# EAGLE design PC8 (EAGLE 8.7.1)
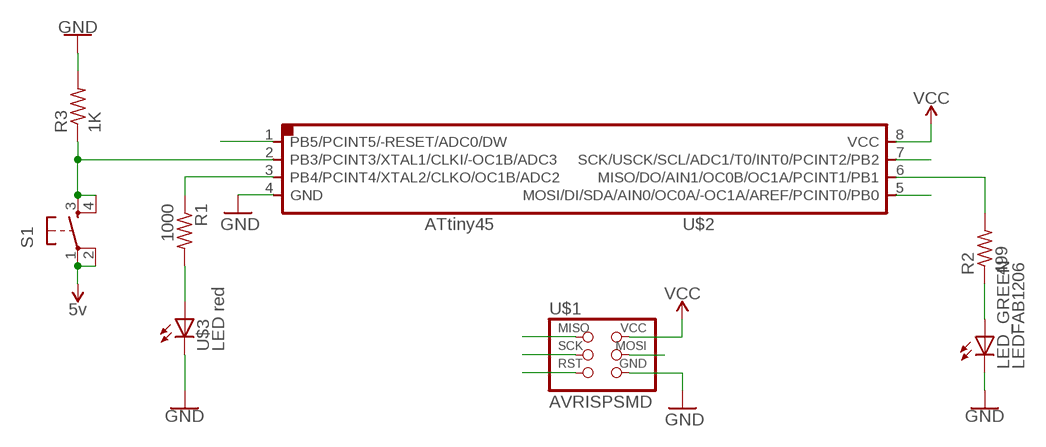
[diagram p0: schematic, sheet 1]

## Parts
LED_GREEN  LEDFAB1206  [LED1206FAB]
R1  1000  RES-US1206FAB  [R1206FAB]
R2  499  RES-US1206FAB  [R1206FAB]
R3  1K  RES-US1206FAB  [R1206FAB]
S1  6MM_SWITCH6MM_SWITCH  [6MM_SWITCH]
U$1  AVRISPSMD  [2X03SMD]
U$2  ATTINY45SI  [SOIC8]
U$3  LED red  LEDFAB1206  [LED1206FAB]

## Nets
GND: LED_GREEN.2(C) R3.2 U$1.6(GND) U$2.4(GND) U$3.2(C)
MISO: R2.2 U$1.1(MISO) U$2.6(MISO/DO/AIN1/OC0B/OC1A/PCINT1/PB1)
MOSI: U$1.4(MOSI) U$2.5(MOSI/DI/SDA/AIN0/OC0A/-OC1A/AREF/PCINT0/PB0)
N$1: R3.1 S1.3(S) S1.4(S1) U$2.2(PB3/PCINT3/XTAL1/CLKI/-OC1B/ADC3)
N$2: R1.1 U$2.3(PB4/PCINT4/XTAL2/CLKO/OC1B/ADC2)
N$3: R1.2 U$3.1(A)
N$4: LED_GREEN.1(A) R2.1
RST: U$1.5(RST) U$2.1(PB5/PCINT5/-RESET/ADC0/DW)
SCK: U$1.3(SCK) U$2.7(SCK/USCK/SCL/ADC1/T0/INT0/PCINT2/PB2)
VCC: S1.1(P) S1.2(P1) U$1.2(VCC) U$2.8(VCC) ; supply symbol labelled 5v

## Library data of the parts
LED_GREEN U$3 = fab (1):LED: LED
R1 R2 = fab:RES-US: Resistor (US Symbol)
R3 = fab (1):RES-US: Resistor (US Symbol)
S1 = fab:6MM_SWITCH: OMRON SWITCH
U$1 = fab:AVRISP
U$2 = fab:ATTINY45

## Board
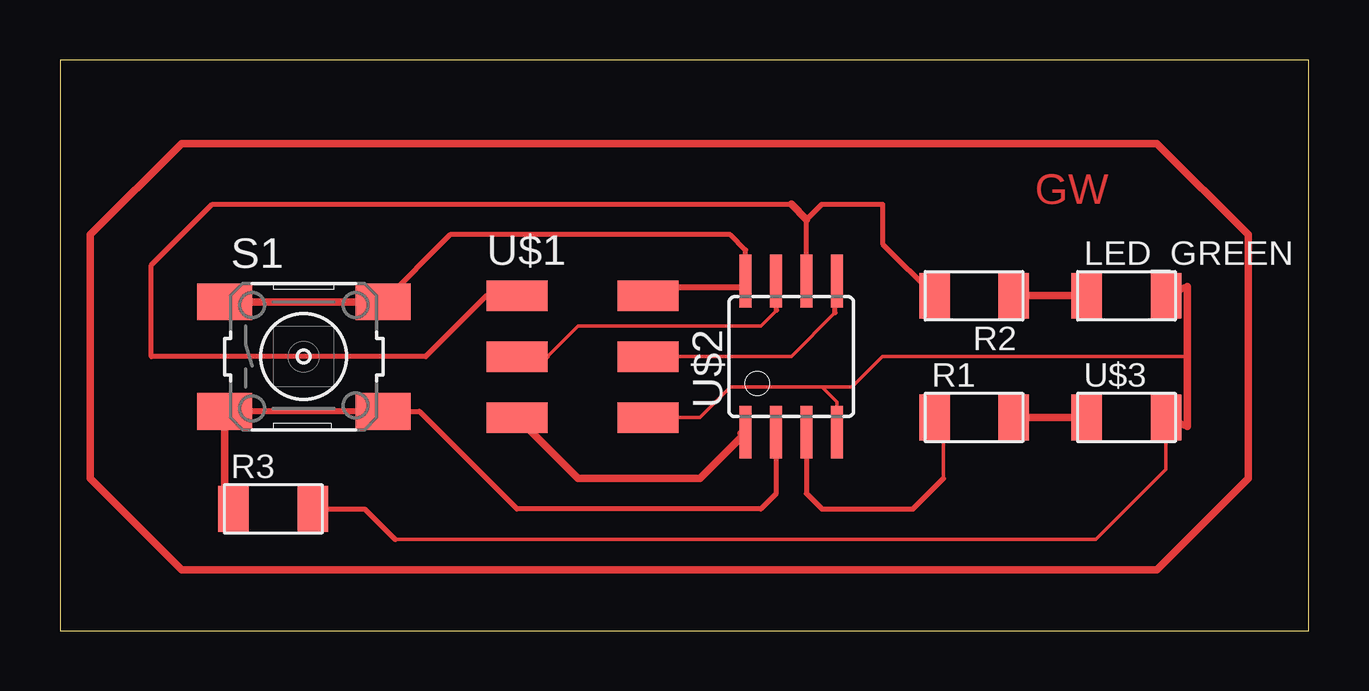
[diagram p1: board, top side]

Size 52.05 x 23.8 mm. Coordinates in mm from the lower left corner, seen from the top.
Outline: 0,0 52.05,0 52.05,23.8 0,23.8 0,0
Copper layers (1*16): Top 0.035mm / dielectric 1.5mm / Bottom 0.035mm
Design rules "default *": minimum track width 10mil, minimum drill 0.35mm, track to track 14mil, track to pad 14mil, pad to pad 14mil, via to via 6mil, smd to smd 14mil, copper to edge 40mil, drill to drill 6mil, minimum pad ring 10mil, minimum via ring 8mil, stop-mask expansion 4mil, vias tented up to drill 0mil, thermal gap 10mil

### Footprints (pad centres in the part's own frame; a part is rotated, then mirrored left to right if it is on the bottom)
LED1206FAB = smd 1.27 x 1.905: 1 -1.651,0; 2 1.651,0
R1206FAB = smd 1.27 x 1.905: 1 -1.651,0; 2 1.651,0
6MM_SWITCH = smd 2.286 x 1.524: 1 -3.302,2.286; 2 3.302,2.286; 3 -3.302,-2.286; 4 3.302,-2.286
2X03SMD = smd 2.54 x 1.27: 1 -2.54,2.54; 2 2.92,2.54; 3 -2.54,0; 4 2.92,0; 5 -2.54,-2.54; 6 2.92,-2.54
SOIC8 = smd 0.5 x 2.2: 1 -1.905,-3.154; 2 -0.645,-3.154; 3 0.625,-3.154; 4 1.895,-3.154; 5 1.905,3.154; 6 0.635,3.154; 7 -0.635,3.154; 8 -1.905,3.154

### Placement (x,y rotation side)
LED_GREEN  44.45,13.97 0 top
R1  38.1,8.89 0 top
R2  38.1,13.97 180 top
R3  [R1206FAB]  8.89,5.08 0 top
S1  10.16,11.43 0 top
U$1  21.59,11.43 0 top
U$2  30.48,11.43 0 top
U$3  44.45,8.89 0 top

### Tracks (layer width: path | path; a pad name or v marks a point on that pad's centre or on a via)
GND
  Top 0.152: 13.97,3.81 43.18,3.81 46.1,6.73 U$3.2 | 46.99,11.43 34.29,11.43 33.02,10.16 31.75,10.16 | U$1.6 26.67,8.89 27.94,10.16 31.75,10.16 | U$2.4 32.38,9.53 31.75,10.16
  Top 0.203: R3.2 12.7,5.08 13.97,3.81
  Top 0.254: 24.69,9.14 U$1.6
  Top 0.305: LED_GREEN.2 46.99,14.35 46.99,11.43 46.99,8.51 U$3.2
MISO
  Top 0.203: U$1.1 17.78,13.97 15.24,11.43 3.81,11.43 3.81,15.24 6.35,17.78 30.48,17.78 | R2.2 34.29,16.13 34.29,17.78 31.75,17.78 31.11,17.14 U$2.6
  Top 0.305: 31.11,17.14 30.48,17.78
MOSI
  Top 0.152: U$1.4 30.48,11.43 32.31,13.26
  Top 0.203: 32.31,13.26 32.31,13.97
  Top 0.254: 32.31,13.72 32.31,13.97 32.31,14.33 U$2.5 | 24.69,11.58 U$1.4
N$1
  Top 0.203: S1.4 14.99,9.14 19.05,5.08 29.21,5.08 29.84,5.71 U$2.2
  Top 0.254: S1.4 S1.3
  Top 0.305: S1.3 6.86,5.46 R3.1
N$2
  Top 0.152: 36.83,6.35 36.83,8.51 R1.1
  Top 0.203: U$2.3 31.11,5.72 31.75,5.08 35.56,5.08 36.83,6.35
N$3
  Top 0.305: R1.2 U$3.1
N$4
  Top 0.305: R2.1 LED_GREEN.1
RST
  Top 0.254: 28.35,8.23 U$2.1 | 19.2,8.84 U$1.5
  Top 0.305: U$1.5 21.59,6.35 26.67,6.35 28.57,8.26 U$2.1
S$1
  Top 0.305: 1.27,16.51 5.08,20.32 45.72,20.32 49.53,16.51 49.53,6.35 45.72,2.54 30.48,2.54 5.08,2.54 1.27,6.35 1.27,16.51
SCK
  Top 0.152: 20.32,11.43 21.59,12.7 29.21,12.7 29.87,13.36
  Top 0.203: U$1.3 20.32,11.43 | 29.87,13.36 29.87,13.97
  Top 0.254: 29.87,13.72 29.87,13.97 29.87,14.33 U$2.7
VCC
  Top 0.203: S1.2 16.26,16.51 27.94,16.51 28.57,15.87 U$2.8
  Top 0.254: U$2.8 28.35,14.33 24.99,14.33 24.69,14.02 U$1.2 24.38,14.02
  Top 0.305: S1.2 14,13.87 13.85,13.72 S1.1

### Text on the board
Top: GW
